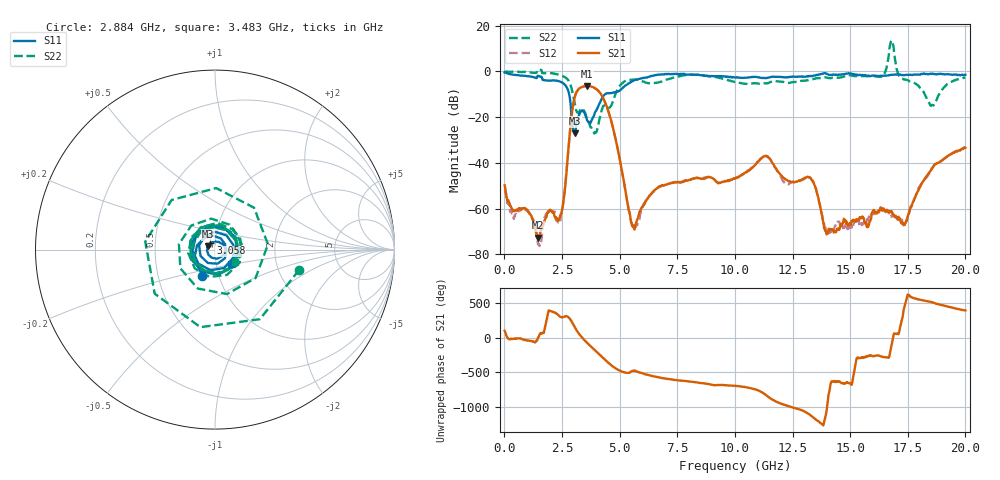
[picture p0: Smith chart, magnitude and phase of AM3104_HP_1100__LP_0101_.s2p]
!Created with skrf (http://scikit-rf.org).
# Hz S RI R 50.0
!freq ReS11 ImS11 ReS21 ImS21 ReS12 ImS12 ReS22 ImS22
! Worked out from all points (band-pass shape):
!   1601 points, 10 MHz to 20 GHz, reference 50 ohm
!   highest |S21| = -6.31 dB at 3.571 GHz (marker M1); lowest = -72.7 dB at 1.459 GHz (marker M2)
!   |S21| within 3 dB of the highest: 3.116 GHz to 4.147 GHz (1.031 GHz wide, 28.4 % of centre)
!   lowest |S11| = -27.1 dB at 3.046 GHz (marker M3), VSWR 1.09, Z = 46.1 + j1.61 ohm
!   |S11| at or under -10 dB: 2.811 GHz to 4.359 GHz (1.548 GHz wide, 43.2 % of centre)
!   |S22| runs from -27.1 to 13.6 dB; largest |S21 - S12| = 0.024
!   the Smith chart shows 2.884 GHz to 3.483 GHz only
!   S11 on the Smith chart (normalised r, x): 2.884 GHz: 0.83, -0.25; 3.058 GHz: 0.95, +0.07; 3.483 GHz: 1.18, -0.20
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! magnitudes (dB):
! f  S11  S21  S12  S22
! 10 MHz  -0.4  -49.8  -51.5  -0.1
! 1.459 GHz  -1.9  -72.7  -75.7  0.8
! 2.434 GHz  -4.5  -62.7  -65.2  -1.7
! 2.884 GHz  -15.8  -22.4  -22.5  -6.3
! 3.046 GHz  -27.1  -11.5  -11.5  -13.8
! 3.058 GHz  -27.1  -11.0  -11.0  -14.5
! 3.346 GHz  -17.3  -6.9  -7.0  -16.3
! 3.483 GHz  -18.2  -6.5  -6.5  -17.6
! 3.571 GHz  -20.7  -6.3  -6.4  -20.1
! 3.933 GHz  -17.8  -7.3  -7.3  -26.7
! 4.508 GHz  -9.5  -17.3  -17.4  -15.8
! 5.582 GHz  -4.1  -67.7  -67.3  -3.6
! 6.682 GHz  -1.4  -50.5  -50.9  -4.8
! 10.01 GHz  -2.7  -46.9  -46.9  -4.6
! 11.33 GHz  -2.9  -37.0  -37.3  -5.2
! 13.34 GHz  -2.1  -47.5  -47.5  -3.5
! 13.97 GHz  -1.0  -70.4  -69.9  -2.7
! 16.35 GHz  -1.9  -60.3  -61.6  -2.3
! 16.68 GHz  -1.6  -61.4  -62.1  7.1
! 17.36 GHz  -1.6  -67.1  -66.1  -3.5
! 18.54 GHz  -1.0  -42.5  -42.6  -14.7
! 20 GHz  -1.4  -33.4  -33.0  -2.7
